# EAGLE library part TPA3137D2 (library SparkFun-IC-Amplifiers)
6W Class D audio amplifier (Stereo)
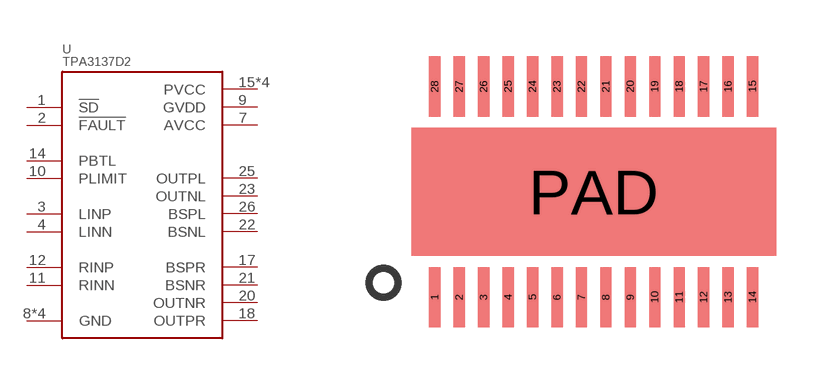
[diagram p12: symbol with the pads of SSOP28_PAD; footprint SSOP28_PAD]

Designator prefix U

## TPA3137D2  [SSOP28_PAD]
1  !SD
2  !FAULT
3  LINP
4  LINN
7  AVCC
8  GND
9  GVDD
10  PLIMIT
11  RINN
12  RINP
14  PBTL
15  PVCC
16  PVCC
17  BSPR
18  OUTPR
19  GND
20  OUTNR
21  BSNR
22  BSNL
23  OUTNL
24  GND
25  OUTPL
26  BSPL
27  PVCC
28  PVCC
PAD  GND

## Footprint SSOP28_PAD (pad centres in mm)
smd 0.3 x 1.6: 1 -4.225,-2.8; 2 -3.575,-2.8; 3 -2.925,-2.8; 4 -2.275,-2.8; 5 -1.625,-2.8; 6 -0.975,-2.8; 7 -0.325,-2.8; 8 0.325,-2.8; 9 0.975,-2.8; 10 1.625,-2.8; 11 2.275,-2.8; 12 2.925,-2.8; 13 3.575,-2.8; 14 4.225,-2.8; 15 4.225,2.8; 16 3.575,2.8; 17 2.925,2.8; 18 2.275,2.8; 19 1.625,2.8; 20 0.975,2.8; 21 0.325,2.8; 22 -0.325,2.8; 23 -0.975,2.8; 24 -1.625,2.8; 25 -2.275,2.8; 26 -2.925,2.8; 27 -3.575,2.8; 28 -4.225,2.8
smd 9.7 x 3.4: PAD 0,0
